//{{V2}}
FUNCTION_BLOCK FB54
TITLE=Get Velocity Is
//*****************************************************************************
//* maxon motor ag
//* R&D
//* all rights reserved
//*****************************************************************************
//* Summary:  Read actual value of velocity
//*
//* Remarks:
//*
//* Created under: STEP7 REV5.2+SP1
//*****************************************************************************
//* History:
//* 19.05.2004 | INA   first release
//*
//*
//*****************************************************************************
//


AUTHOR:INA
FAMILY:MotionIn
NAME:GetVelIs
VERSION:00.01


VAR_INPUT
       Read:BOOL //A rising edge start the command
       NodeID:BYTE //Adress of the maxon device
END_VAR

VAR_OUTPUT
       Done:BOOL //Data valid flag is TRUE if data were available
       Err:BOOL //Error flag is TRUE if an Error has occured, see ErrNo for more details
       ErrNo:DINT //Contains detailed error information
       VelocityIs:DINT //Velocity actual value
END_VAR

VAR_IN_OUT
END_VAR

VAR
       xEdgeMerker:BOOL //Edge Merker
       xEdgeFlag:BOOL //Edge Flag
       xStep:INT
END_VAR

VAR_TEMP
END_VAR
BEGIN

NETWORK
TITLE= Activate the service function
//{{a}}
//

// SDO Read "Get Velocity is"

       U    #Read
       FP   #xEdgeFlag                   // recognize a positiv edge of the Read signal
       =    #xEdgeMerker                 // and set the xEdgeMerker for one cycle to true

       L    #xStep
       L    0
       ==I
       U    #xEdgeMerker
       SPB  nstp                         // iStep = 1 -> fnc1

       L    #xStep                       // jump list
       SPL  List
       SPA  rdef
       SPA  fnc1
       SPA  fncE
List  :SPA  rdef

rdef  :NOP  0
       R    #Done                        // reset Done
       R    #Err                         // reset Error
       L    0
       T    #xStep                       // iStep = 0
       SPA  end

fnc1  :NOP  0
       CALL FC1
         NodeID:=#NodeID
         Index:=DW#16#00002028
         SubIndex:=DW#16#00000000        // Velocity actual value averaged
         RET_VAL:=#Done
         Err:=#Err
         ErrNo:=#ErrNo

       L    DB219.DBD10
       T    #VelocityIs

fncE  :NOP  0
       L    0
       T    #xStep
       SPA  end

nstp  :NOP  0
       L    #xStep
       INC            1
       T    #xStep

end   :NOP  0
END_FUNCTION_BLOCK
